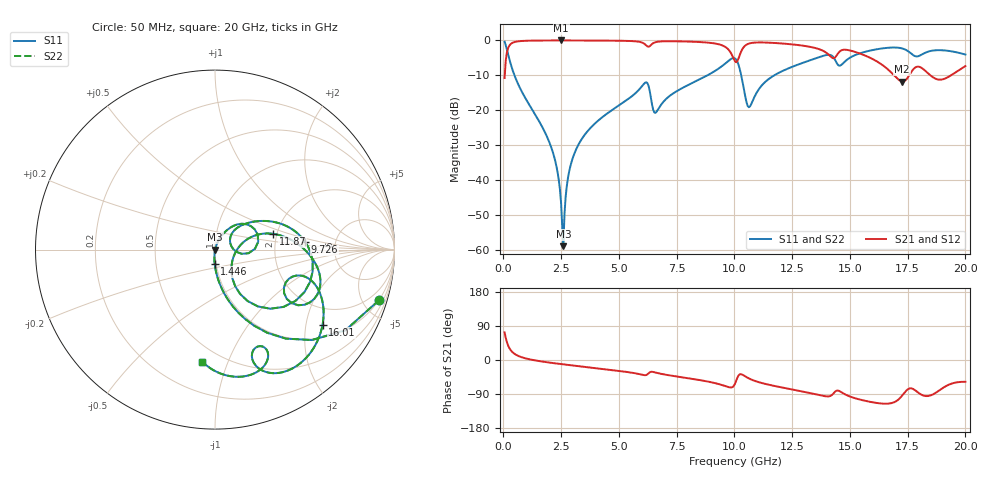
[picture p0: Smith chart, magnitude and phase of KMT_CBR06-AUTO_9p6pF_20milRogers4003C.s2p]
! Data measured by Modelithics Inc. support@modelithics.com 813-866-6335
! KEMET CBR06-AUTO 9.6pF, Pad Width= 0.851mm, Pad Length= 0.64mm, Pad Gap= 0.62mm, 20mil Rogers 4003C substrate Data, January 2022
# hz S ma R 50
! 2 Port Network Data from SP1.SP block
! freq  magS11  angS11  magS21  angS21  magS12  angS12  magS22  angS22
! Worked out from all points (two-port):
!   401 points, 50 MHz to 20 GHz, reference 50 ohm
!   highest |S21| = -0.01 dB at 2.494 GHz (marker M1); lowest = -11.8 dB at 17.26 GHz (marker M2)
!   |S21| within 3 dB of the highest: 167.3 MHz to 9.789 GHz (9.621 GHz wide, 193 % of centre); 10.3 GHz to 13.85 GHz (3.546 GHz wide, 29.4 % of centre)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
!   lowest |S11| = -58.9 dB at 2.594 GHz (marker M3), VSWR 1.00, Z = 50.1 + j0.0391 ohm
!   |S11| at or under -10 dB: 478.1 MHz to 8.827 GHz (8.349 GHz wide, 179 % of centre); 10.29 GHz to 11.72 GHz (1.428 GHz wide, 13 % of centre)
!   |S22| runs from -58.9 to -0.4 dB; largest |S21 - S12| = 0
!   S11 on the Smith chart (normalised r, x): 50 MHz: 0.98, -6.50; 1.446 GHz: 0.98, -0.16; 9.726 GHz: 3.00, +0.34; 11.87 GHz: 1.92, +0.38; 16.01 GHz: 1.38, -2.49; 20 GHz: 0.39, -0.81
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5e7  0.9567 -17.1  0.2906 72.9  0.2906 72.9  0.9567 -17.1
4.49e8  0.3354 -72.3  0.9415 17.6  0.9415 17.6  0.3354 -72.3
1.4465e9  0.07917 -91.3  0.996 -1.9  0.996 -1.9  0.07917 -91.3
2.194625e9  0.02169 -96.1  0.9988 -8.5  0.9988 -8.5  0.02169 -96.1
2.493875e9  0.004771 -89.3  0.999 -10.8  0.999 -10.8  0.004771 -89.3
2.593625e9  0.001138 20.1  0.9989 -11.5  0.9989 -11.5  0.001138 20.1
2.892875e9  0.01562 72.5  0.9987 -13.7  0.9987 -13.7  0.01562 72.5
3.391625e9  0.03891 71.1  0.998 -17.2  0.998 -17.2  0.03891 71.1
6.13475e9  0.2485 26.9  0.8761 -40.1  0.8761 -40.1  0.2485 26.9
6.73325e9  0.1081 38.0  0.9634 -35.4  0.9634 -35.4  0.1081 38.0
9.72575e9  0.5049 4.8  0.7493 -71.3  0.7493 -71.3  0.5049 4.8
1.0025e10  0.5519 -25.4  0.5031 -62.7  0.5031 -62.7  0.5519 -25.4
1.06235e10  0.1107 -21.1  0.9 -48.5  0.9 -48.5  0.1107 -21.1
1.187038e10  0.3371 15.1  0.9136 -70.2  0.9136 -70.2  0.3371 15.1
1.336662e10  0.5326 -3.8  0.798 -88.5  0.798 -88.5  0.5326 -3.8
1.451375e10  0.4379 -28.7  0.6705 -81.2  0.6705 -81.2  0.4379 -28.7
1.601e10  0.7314 -35.0  0.5358 -111.9  0.5358 -111.9  0.7314 -35.0
1.670825e10  0.7876 -49.5  0.3688 -114.8  0.3688 -114.8  0.7876 -49.5
1.725688e10  0.7691 -63.5  0.2578 -94.2  0.2578 -94.2  0.7691 -63.5
1.790525e10  0.5901 -66.1  0.4207 -83.6  0.4207 -83.6  0.5901 -66.1
1.890275e10  0.7251 -76.2  0.2745 -78.9  0.2745 -78.9  0.7251 -76.2
2e10  0.6283 -96.4  0.4292 -57.5  0.4292 -57.5  0.6283 -96.4
